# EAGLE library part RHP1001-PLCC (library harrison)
Intan Technologies RHP1001 patch clamp chip (PLCC-44 package)
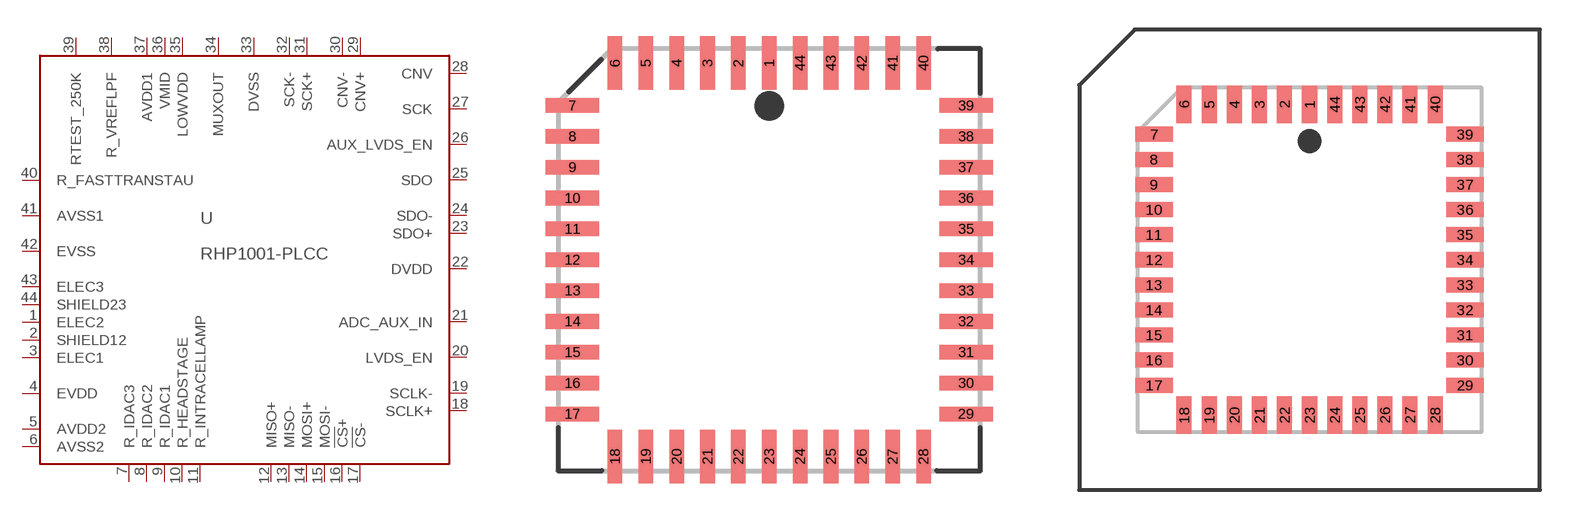
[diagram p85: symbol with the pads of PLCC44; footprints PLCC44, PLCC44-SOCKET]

Designator prefix U

## RHP1001-PLCC  [PLCC44]
1  ELEC2  in
2  SHIELD12  pas
3  ELEC1  in
4  EVDD  pwr
5  AVDD2  pwr
6  AVSS2  pwr
7  R_IDAC3  pas
8  R_IDAC2  pas
9  R_IDAC1  pas
10  R_HEADSTAGE  pas
11  R_INTRACELLAMP  pas
12  MISO+  out
13  MISO-  out
14  MOSI+  in
15  MOSI-  in
16  !CS!+  in
17  !CS!-  in
18  SCLK+  in
19  SCLK-  in
20  LVDS_EN  in
21  ADC_AUX_IN  in
22  DVDD  pwr
23  SDO+  out
24  SDO-  out
25  SDO  in
26  AUX_LVDS_EN  in
27  SCK  out
28  CNV  out
29  CNV+  in
30  CNV-  in
31  SCK+  in
32  SCK-  in
33  DVSS  pwr
34  MUXOUT  out
35  LOWVDD  pwr
36  VMID  pwr
37  AVDD1  pwr
38  R_VREFLPF  pas
39  RTEST_250K  pas
40  R_FASTTRANSTAU  pas
41  AVSS1  pwr
42  EVSS  pwr
43  ELEC3  in
44  SHIELD23  pas

## RHP1001-PLCC-SOCKET  [PLCC44-SOCKET]
Pads as for PLCC44

## Footprint PLCC44 (pad centres in mm)
smd 0.6 x 2.2: 1 0,8.1; 2 -1.27,8.1; 3 -2.54,8.1; 4 -3.81,8.1; 5 -5.08,8.1; 6 -6.35,8.1; 18 -6.35,-8.1; 19 -5.08,-8.1; 20 -3.81,-8.1; 21 -2.54,-8.1; 22 -1.27,-8.1; 23 0,-8.1; 24 1.27,-8.1; 25 2.54,-8.1; 26 3.81,-8.1; 27 5.08,-8.1; 28 6.35,-8.1; 40 6.35,8.1; 41 5.08,8.1; 42 3.81,8.1; 43 2.54,8.1; 44 1.27,8.1
smd 2.2 x 0.6: 7 -8.1,6.35; 8 -8.1,5.08; 9 -8.1,3.81; 10 -8.1,2.54; 11 -8.1,1.27; 12 -8.1,0; 13 -8.1,-1.27; 14 -8.1,-2.54; 15 -8.1,-3.81; 16 -8.1,-5.08; 17 -8.1,-6.35; 29 8.1,-6.35; 30 8.1,-5.08; 31 8.1,-3.81; 32 8.1,-2.54; 33 8.1,-1.27; 34 8.1,0; 35 8.1,1.27; 36 8.1,2.54; 37 8.1,3.81; 38 8.1,5.08; 39 8.1,6.35

## Footprint PLCC44-SOCKET (pad centres in mm)
PLCC SMD socket - DigiKey P/N AE10071-ND
smd 0.76 x 1.91: 1 0,7.87; 2 -1.27,7.87; 3 -2.54,7.87; 4 -3.81,7.87; 5 -5.08,7.87; 6 -6.35,7.87; 18 -6.35,-7.87; 19 -5.08,-7.87; 20 -3.81,-7.87; 21 -2.54,-7.87; 22 -1.27,-7.87; 23 0,-7.87; 24 1.27,-7.87; 25 2.54,-7.87; 26 3.81,-7.87; 27 5.08,-7.87; 28 6.35,-7.87; 40 6.35,7.87; 41 5.08,7.87; 42 3.81,7.87; 43 2.54,7.87; 44 1.27,7.87
smd 1.91 x 0.76: 7 -7.87,6.35; 8 -7.87,5.08; 9 -7.87,3.81; 10 -7.87,2.54; 11 -7.87,1.27; 12 -7.87,0; 13 -7.87,-1.27; 14 -7.87,-2.54; 15 -7.87,-3.81; 16 -7.87,-5.08; 17 -7.87,-6.35; 29 7.87,-6.35; 30 7.87,-5.08; 31 7.87,-3.81; 32 7.87,-2.54; 33 7.87,-1.27; 34 7.87,0; 35 7.87,1.27; 36 7.87,2.54; 37 7.87,3.81; 38 7.87,5.08; 39 7.87,6.35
